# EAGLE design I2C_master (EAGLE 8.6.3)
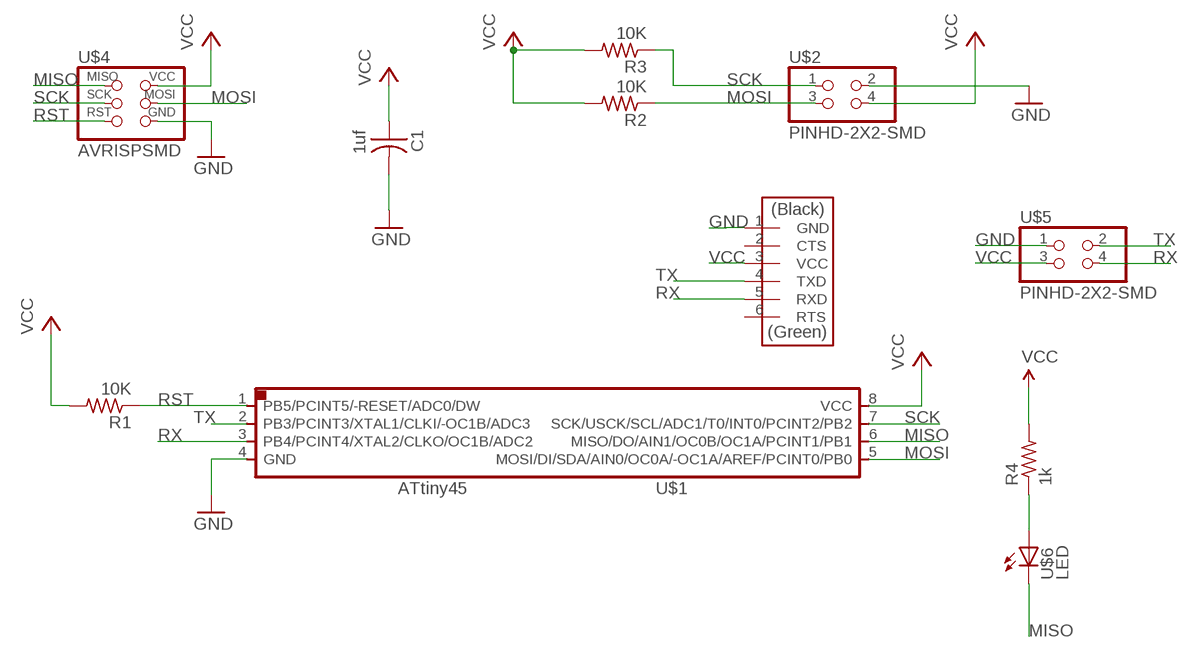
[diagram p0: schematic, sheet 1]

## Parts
C1  1uf  CAP-US1206FAB  [C1206FAB]
R1  10K  RES-US1206FAB  [R1206FAB]
R2  10K  RES-US1206FAB  [R1206FAB]
R3  10K  RES-US1206FAB  [R1206FAB]
R4  1k  RESISTOR1206  [1206]
U$1  ATTINY45SI  [SOIC8]
U$2  PINHD-2X2-SMD  [2X02SMD]
U$3  FTDI-SMD-HEADER  [1X06SMD]
U$4  AVRISPSMD  [2X03SMD]
U$5  PINHD-2X2-SMD  [2X02SMD]
U$6  LED  [LED1206]

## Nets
GND: C1.2 U$1.4(GND) U$2.2 U$3.1(GND) U$4.6(GND) U$5.1
MISO: U$1.6(MISO/DO/AIN1/OC0B/OC1A/PCINT1/PB1) U$4.1(MISO) U$6.2(C)
MOSI: R2.1 U$1.5(MOSI/DI/SDA/AIN0/OC0A/-OC1A/AREF/PCINT0/PB0) U$2.3 U$4.4(MOSI)
N$3: R4.1 U$6.1(A)
RST: R1.1 U$1.1(PB5/PCINT5/-RESET/ADC0/DW) U$4.5(RST)
RX: U$1.3(PB4/PCINT4/XTAL2/CLKO/OC1B/ADC2) U$3.5(RXD) U$5.4
SCK: R3.1 U$1.7(SCK/USCK/SCL/ADC1/T0/INT0/PCINT2/PB2) U$2.1 U$4.3(SCK)
TX: U$1.2(PB3/PCINT3/XTAL1/CLKI/-OC1B/ADC3) U$3.4(TXD) U$5.2
VCC: C1.1 R1.2 R2.2 R3.2 R4.2 U$1.8(VCC) U$2.4 U$3.3(VCC) U$4.2(VCC) U$5.3
Unconnected: U$3.2(CTS) U$3.6(RTS)

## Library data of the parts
C1 = fab:CAP-US
R1-R3 = fab:RES-US: Resistor (US Symbol)
R4 = FAB_Hello:RESISTOR
U$1 = fab:ATTINY45
U$2 = fab:PINHD-2X2-SMD
U$3 = fab:FTDI-SMD-HEADER
U$4 = fab:AVRISP
U$5 = 01_fab:PINHD-2X2-SMD
U$6 = fab:LED: LED

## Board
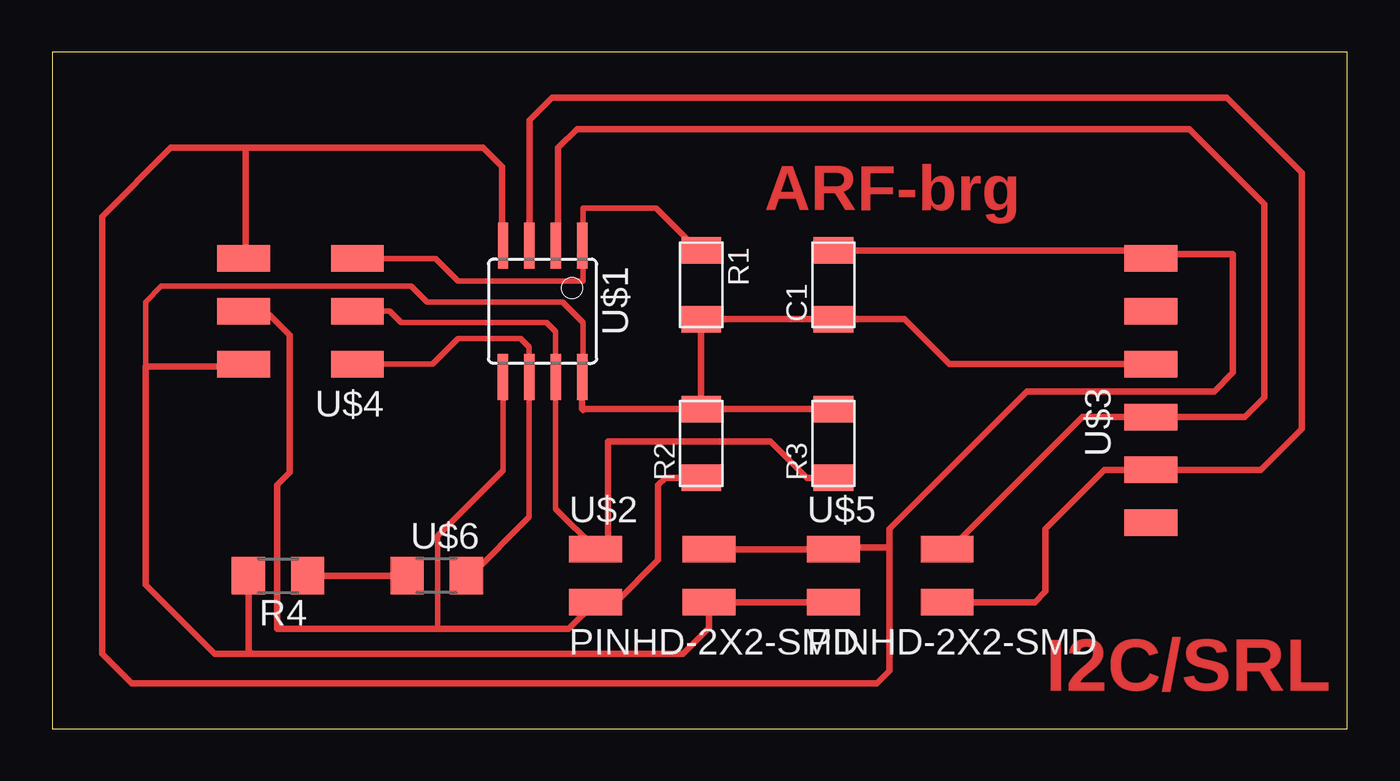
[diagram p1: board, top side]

Size 62.2 x 32.5 mm. Coordinates in mm from the lower left corner, seen from the top.
Outline: 0,0 62.2,0 62.2,32.5 0,32.5 0,0
Copper layers (1*16): Top 0.035mm / dielectric 1.5mm / Bottom 0.035mm
Design rules "default *": minimum track width 40mm, minimum drill 0.35mm, track to track 6mil, track to pad 6mil, pad to pad 6mil, via to via 6mil, smd to smd 6mil, copper to edge 80mil, drill to drill 6mil, minimum pad ring 10mil, minimum via ring 8mil, stop-mask expansion 4mil, vias tented up to drill 0mil, thermal gap 10mil

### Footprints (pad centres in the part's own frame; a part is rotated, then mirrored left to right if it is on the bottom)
C1206FAB = smd 1.27 x 1.905: 1 -1.651,0; 2 1.651,0
R1206FAB = smd 1.27 x 1.905: 1 -1.651,0; 2 1.651,0
1206 = smd 1.6 x 1.803: 1 -1.422,0; 2 1.422,0
SOIC8 = smd 0.5 x 2.2: 1 -1.905,-3.154; 2 -0.645,-3.154; 3 0.625,-3.154; 4 1.895,-3.154; 5 1.905,3.154; 6 0.635,3.154; 7 -0.635,3.154; 8 -1.905,3.154
2X02SMD = smd 2.54 x 1.27: 1 -2.54,1.27; 2 2.92,1.27; 3 -2.54,-1.27; 4 2.92,-1.27
1X06SMD = smd 2.54 x 1.27: 1 0,6.35; 2 0,3.81; 3 0,1.27; 4 0,-1.27; 5 0,-3.81; 6 0,-6.35
2X03SMD = smd 2.54 x 1.27: 1 -2.54,2.54; 2 2.92,2.54; 3 -2.54,0; 4 2.92,0; 5 -2.54,-2.54; 6 2.92,-2.54
LED1206 = smd 1.6 x 1.803: 1 -1.422,0; 2 1.422,0

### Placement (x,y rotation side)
C1  37.52,21.32 90 top
R1  31.17,21.32 270 top
R2  31.17,13.7 90 top
R3  37.52,13.7 90 top
R4  10.85,7.35 180 top
U$1  23.55,20.05 180 top
U$2  28.63,7.35 0 top
U$3  52.76,16.24 0 top
U$4  12.12,20.05 180 top
U$5  40.06,7.35 0 top
U$6  18.47,7.35 0 top

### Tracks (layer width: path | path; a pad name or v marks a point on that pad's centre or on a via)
GND
  Top 0.305: U$1.4 21.6,23.26 21.6,27 20.7,27.9 9.3,27.9 | 9.3,27.9 5.7,27.9 2.4,24.6 2.4,3.6 3.82,2.18 39.6,2.18 40.2,2.78 40.2,8.4 40.2,8.7 | 40.2,8.7 37.6,8.7 U$5.1 U$2.2 | 52.97,22.8 56.7,22.8 56.7,17.1 55.8,16.2 46.8,16.2 40.2,9.6 40.2,8.7 | 52.97,22.8 52.88,22.71 | U$3.1 52.88,22.71 | 52.97,22.8 53.1,22.93 | U$4.6 9.3,22.69 9.3,27.9 | C1.2 52.63,22.97 52.88,22.71
MISO
  Top 0.254: U$6.2 20.1,7.35 22.91,10.16 U$1.6 22.91,18.34 22.5,18.75 19.5,18.75 18.26,17.51 U$4.1
MOSI
  Top 0.254: U$1.5 21.64,12.39 18.5,9.25 18.5,4.8
  Top 0.305: U$4.4 10.25,20.05 11.4,18.9 11.4,12.3 10.8,11.7 10.8,4.8 18.5,4.8 24.81,4.8 U$2.3 27.08,6.08 29.1,8.1 29.1,11.7 29.45,12.05 R2.1
N$3
  Top 0.305: R4.1 U$6.1
RST
  Top 0.254: U$4.5 18.41,22.59 19.5,21.5 25.5,21.5 25.5,23.16 | U$1.1 25.5,23.25 25.5,25 29,25 31.03,22.97 R1.1
  Top 0.305: 25.5,23.16 U$1.1
RX
  Top 0.305: U$1.3 22.93,29.23 24,30.3 56.4,30.3 60,26.7 60,14.4 58.03,12.43 U$3.5 50.53,12.43 47.7,9.6 47.7,6.6 47.18,6.08 U$5.4
SCK
  Top 0.254: U$4.3 16.2,20.05 16.75,19.5 23.75,19.5 24.18,19.07 U$1.7 24.18,10.56 26.09,8.66 U$2.1
  Top 0.305: U$2.1 26.7,9.23 26.7,13.8 34.5,13.8 36.25,12.05 R3.1
  Top 0.406: 26.09,9.01 U$2.1 27.08,8.62
TX
  Top 0.305: U$1.2 24.3,23.31 24.3,27.9 25.2,28.8 54.6,28.8 58.2,25.2 58.2,15.9 57.27,14.97 U$3.4 49.47,14.97 43.12,8.62 U$5.2
VCC
  Top 0.254: 25.5,16.94 25.5,19.5 24.5,20.5 18,20.5 17.25,21.25 5.25,21.25 4.5,20.5 4.5,17.4
  Top 0.305: U$3.3 43.09,17.51 40.93,19.67 C1.1 R1.2 R2.2 | R3.2 R2.2 | R2.2 25.55,15.35 25.5,15.3 25.45,15.35 U$1.8 25.5,16.94 | 9.6,3.6 7.8,3.6 4.5,6.9 4.5,17.4 9.09,17.4 U$4.2 | 9.6,3.6 30.3,3.6 31.55,4.85 U$2.4 U$5.3 | R4.2 9.43,3.77 9.6,3.6

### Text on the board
Top: ARF-brg | I2C/SRL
